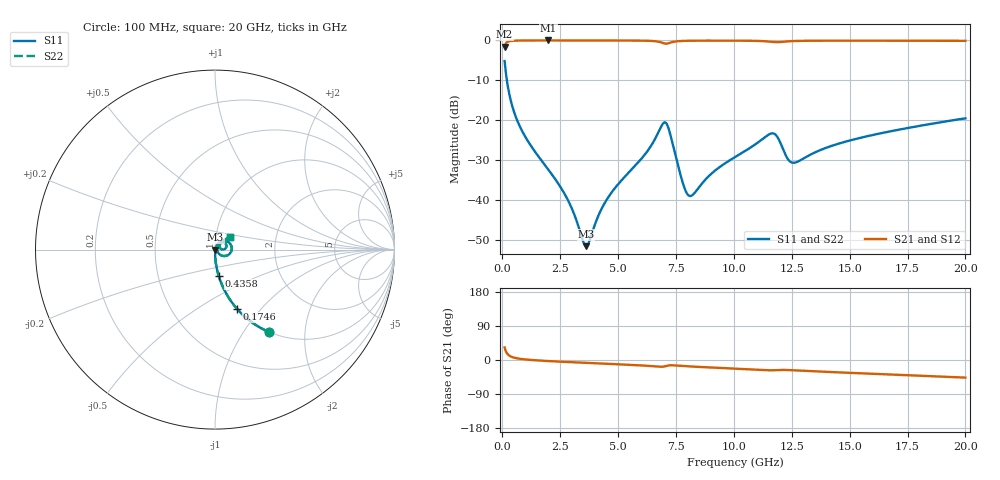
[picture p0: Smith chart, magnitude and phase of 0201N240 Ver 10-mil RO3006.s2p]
# GHz S MA R 50
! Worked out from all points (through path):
!   1601 points, 100 MHz to 20 GHz, reference 50 ohm
!   highest |S21| = -0.02 dB at 1.99 GHz (marker M1); lowest = -1.6 dB at 100 MHz (marker M2)
!   group delay of S21, straight-line fit = 6.87 ps
!   lowest |S11| = -51.6 dB at 3.62 GHz (marker M3), VSWR 1.01, Z = 50.3 - j0.0491 ohm
!   |S11| at or under -10 dB: 197.6 MHz to end of sweep
!   |S22| runs from -51.6 to -5.2 dB; largest |S21 - S12| = 0
!   S11 on the Smith chart (normalised r, x): 100 MHz: 1.00, -1.32; 174.6 MHz: 1.00, -0.75; 435.8 MHz: 1.00, -0.30; 20 GHz: 1.16, +0.16
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0.1  0.5508 -56.7  0.8338 33.2  0.8338 33.2  0.5508 -56.7
0.174625  0.3531 -69.5  0.9347 20.3  0.9347 20.3  0.3531 -69.5
0.4358125  0.1479 -82.0  0.988 7.6  0.988 7.6  0.1479 -82.0
0.970625  0.06345 -87.2  0.9966 1.6  0.9966 1.6  0.06345 -87.2
1.9905  0.02393 -88.3  0.9978 -2.8  0.9978 -2.8  0.02393 -88.3
2.848688  0.00975 -82.0  0.9976 -5.4  0.9976 -5.4  0.00975 -82.0
3.420812  0.003486 -50.5  0.9974 -7.0  0.9974 -7.0  0.003486 -50.5
3.619813  0.002629 -10.7  0.9973 -7.5  0.9973 -7.5  0.002629 -10.7
4.540188  0.0104 62.2  0.9967 -10.0  0.9967 -10.0  0.0104 62.2
6.181938  0.03783 61.9  0.9906 -15.0  0.9906 -15.0  0.03783 61.9
6.741625  0.07049 43.4  0.9637 -17.6  0.9637 -17.6  0.07049 43.4
6.9655  0.09228 16.4  0.9219 -17.4  0.9219 -17.4  0.09228 16.4
7.127187  0.08656 -13.7  0.9133 -14.9  0.9133 -14.9  0.08656 -13.7
7.798813  0.01622 -34.8  0.9844 -15.9  0.9844 -15.9  0.01622 -34.8
8.084875  0.01121 0.5  0.9891 -17.0  0.9891 -17.0  0.01121 0.5
10.05  0.03442 55.3  0.9921 -22.7  0.9921 -22.7  0.03442 55.3
11.65444  0.06831 25.7  0.9569 -27.2  0.9569 -27.2  0.06831 25.7
11.87831  0.06163 9.0  0.9489 -26.5  0.9489 -26.5  0.06163 9.0
12.47531  0.02967 17.3  0.9782 -26.9  0.9782 -26.9  0.02967 17.3
13.37081  0.03772 45.6  0.9894 -29.6  0.9894 -29.6  0.03772 45.6
16.69162  0.07176 46.6  0.9905 -38.1  0.9905 -38.1  0.07176 46.6
20  0.1055 39.8  0.9871 -46.5  0.9871 -46.5  0.1055 39.8
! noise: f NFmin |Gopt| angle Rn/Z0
0.1  0.0006189  0.9307  0.3066  0.001985
2.301  0.004269  0.7862  4.835  0.004098
4.515  0.007489  0.7644  9.393  0.006415
6.729  0.02961  0.9045  13.98  0.06701
8.943  0.01556  0.7761  18.51  0.01385
11.14  0.02628  0.831  22.96  0.03148
13.36  0.02232  0.7712  27.39  0.01879
15.57  0.02006  0.7154  31.65  0.01291
17.79  0.02121  0.6987  35.86  0.01251
20  0.02283  0.6905  40  0.01273
